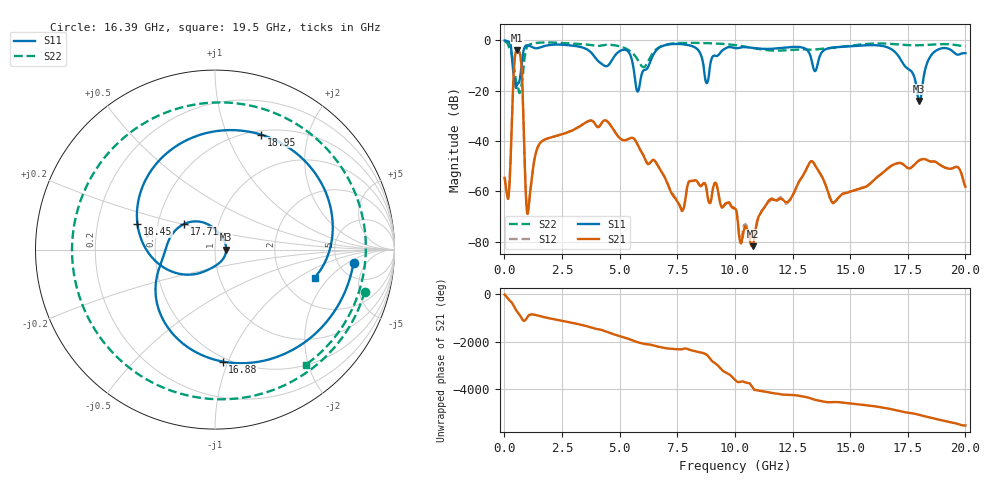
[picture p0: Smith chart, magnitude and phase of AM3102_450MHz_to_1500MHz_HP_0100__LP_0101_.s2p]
!Agilent Technologies,E8364B,MY43040894,A.07.50.67
!Agilent E8364B: A.07.50.67
!Date: Thursday, January 11, 2018 05:36:24
!Correction: S11(Full 2 Port(1,2))
!S21(Full 2 Port(1,2))
!S12(Full 2 Port(1,2))
!S22(Full 2 Port(1,2))
!S2P File: Measurements: S11, S21, S12, S22:
# Hz S  dB  R 50
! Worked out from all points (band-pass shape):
!   1601 points, 10 MHz to 20 GHz, reference 50 ohm
!   highest |S21| = -3.86 dB at 559.7 MHz (marker M1); lowest = -81.7 dB at 10.77 GHz (marker M2)
!   |S21| within 3 dB of the highest: 453.5 MHz to 704.3 MHz (250.8 MHz wide, 43.3 % of centre)
!   lowest |S11| = -24.0 dB at 18 GHz (marker M3), VSWR 1.13, Z = 56.7 - j0.004 ohm
!   |S11| at or under -10 dB: 356 MHz to 746.7 MHz (390.7 MHz wide, 70.9 % of centre); 5.584 GHz to 6.262 GHz (678.5 MHz wide, 11.5 % of centre); 17.35 GHz to 18.3 GHz (948.5 MHz wide, 5.32 % of centre)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
!   |S22| runs from -20.9 to -0.4 dB; largest |S21 - S12| = 0.0026
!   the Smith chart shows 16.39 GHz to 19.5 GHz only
!   S11 on the Smith chart (normalised r, x): 16.39 GHz: 6.96, -2.54; 16.88 GHz: 0.47, -0.96; 17.71 GHz: 0.68, +0.21; 18.45 GHz: 0.38, +0.14; 18.95 GHz: 0.54, +1.33; 19.5 GHz: 3.01, -1.40
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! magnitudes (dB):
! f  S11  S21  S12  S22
! 10 MHz  -0.1  -54.6  -54.5  -0.4
! 197.4 MHz  -0.7  -60.6  -59.0  -2.6
! 559.7 MHz  -17.3  -3.9  -3.9  -18.0
! 722.1 MHz  -11.8  -8.2  -8.2  -19.0
! 1.022 GHz  -2.0  -68.6  -67.9  -2.2
! 1.534 GHz  -2.9  -41.0  -41.0  -0.9
! 3.346 GHz  -2.7  -33.7  -33.7  -1.5
! 5.782 GHz  -20.3  -41.5  -41.5  -7.7
! 6.682 GHz  -3.1  -50.1  -50.1  -3.0
! 10.01 GHz  -3.1  -66.8  -66.2  -1.9
! 10.77 GHz  -3.0  -81.7  -81.0  -3.0
! 13.34 GHz  -8.4  -48.0  -48.0  -3.8
! 14.28 GHz  -2.8  -64.6  -64.1  -3.0
! 16.39 GHz  -2.2  -52.7  -52.8  -1.2
! 16.68 GHz  -3.0  -50.5  -50.5  -1.3
! 16.88 GHz  -4.1  -49.4  -49.4  -1.5
! 17.71 GHz  -13.0  -50.1  -50.0  -2.0
! 18 GHz  -24.0  -47.7  -47.6  -2.0
! 18.45 GHz  -6.8  -48.0  -48.0  -1.8
! 18.95 GHz  -3.2  -49.8  -49.7  -1.5
! 19.5 GHz  -4.8  -50.5  -50.6  -1.8
! 20 GHz  -5.1  -58.2  -58.0  -2.4
